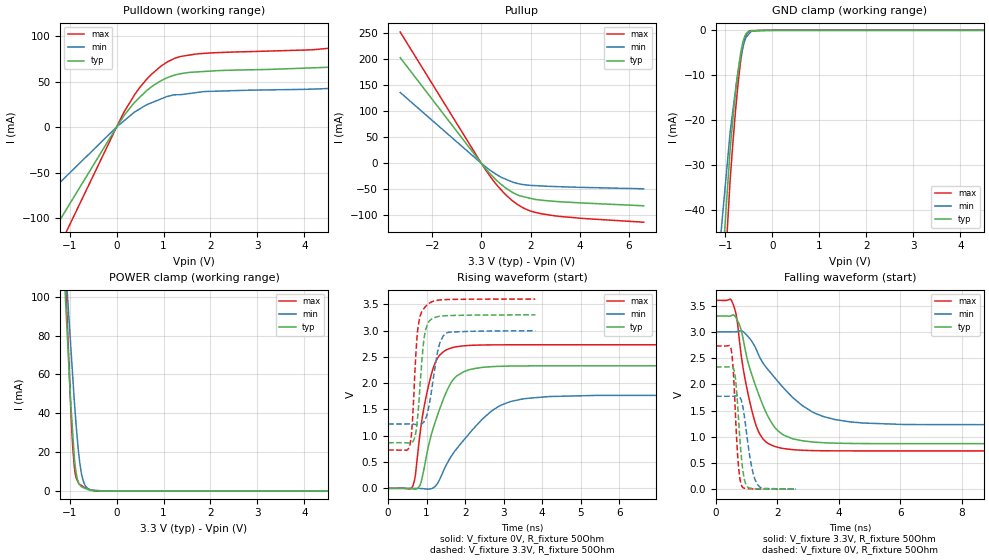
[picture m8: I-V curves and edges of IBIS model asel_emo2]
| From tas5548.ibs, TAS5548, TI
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|   asel_emo2 Model
[Model]   asel_emo2
Model_type   I/O
Polarity   Non-Inverting
Enable   Active-Low
Vinl = 0.8
Vinh = 2.0
Vmeas = 1.65
Vref = 1.65
Cref = 2pF
Rref = 50
|   typ   min   max
|   (nom PVT)   (fast PVT)   (slow PVT)
|C_comp from frequency sweep method (F=50MHz)
|Average
|C_comp   3.022e-12   2.885e-12   3.227e-12
|ON state : BUFFER OUTPUT TURNED HIGH
|C_comp   4.084e-12   3.837e-12   4.481e-12
|OFF state: BUFFER IN HIGH IMPEDANCE
|C_comp   1.959e-12   1.934e-12   1.973e-12
|C_comp from LC tank measurement(L=1nH)
|Average
|Resonant Frequency(Hz)   3.780e+09   3.820e+09   3.745e+09
C_comp   1.788e-12   1.746e-12   1.824e-12
|ON state : BUFFER OUTPUT TURNED HIGH
|Resonant Frequency(Hz)   3.590e+09   3.670e+09   3.540e+09
|C_comp   1.967e-12   1.883e-12   2.023e-12
|OFF state: BUFFER IN HIGH IMPEDANCE
|Resonant Frequency(Hz)   3.970e+09   3.970e+09   3.950e+09
|C_comp   1.609e-12   1.609e-12   1.625e-12
| Where nom  PVT is Nominal Process, 3.3V, 27C
|   Fast PVT is Strong Process,  3.6V, 0C
|   Slow PVT is Weak Process,   3V, 125C
[Voltage Range]   3.3   3   3.6
|Ambient Temperature   27   125   0
|Junction Temperature
[Temperature Range]   27   125   0
[Pullup Reference]   3.3   3   3.6
[Pulldown Reference]   0   0   0
[Power Clamp Reference]   3.3   3   3.6
[GND Clamp Reference]   0   0   0
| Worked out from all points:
|   slope of the pulldown table from 0 to 0.495 V, typ, clamps not added: 15.1 ohm
|   slope of the pullup table from 0 to 0.495 V, typ, clamps not added: 18.5 ohm
|   GND clamp passes 1 mA (typ) near -0.57 V on its own axis
|   POWER clamp passes 1 mA (typ) near -0.64 V on its own axis
|   falling waveform, V_fixture 3.3V, R_fixture 50Ohm: 20-80 % time 825ps typ, 1.52ns min, 530ps max; typ from 3.3 V to 0.868 V
|   rising waveform, V_fixture 0V, R_fixture 50Ohm: 20-80 % time 574ps typ, 1.15ns min, 377ps max; typ from 0 V to 2.33 V
|   rising waveform, V_fixture 3.3V, R_fixture 50Ohm: 20-80 % time 160ps typ, 234ps min, 137ps max; typ from 0.868 V to 3.3 V
|   falling waveform, V_fixture 0V, R_fixture 50Ohm: 20-80 % time 180ps typ, 271ps min, 146ps max; typ from 2.33 V to 0.001 V
[Pulldown]
|   Voltage   I(typ)   I(min)   I(max)
-3.3V     -279.4mA   -166.6mA   -355.3mA
-3mV      -254uA     -151.5uA   -323uA
396mV     27.87mA    16.95mA    36.54mA
633.6mV   39.82mA    24.42mA    52.19mA
939.6mV   50.83mA    30.86mA    66.82mA
1.246V    57.38mA    35.55mA    75.8mA
2.012V    61.64mA    39.34mA    81.57mA
4.496V    65.86mA    42.46mA    86.57mA
5.148V    71.83mA    45.78mA    94.35mA
5.683V    83.14mA    53.28mA    109.3mA
6.158V    100.8mA    61.11mA    132.7mA
6.6V      125.8mA    68.39mA    165.9mA
[GND Clamp]
|   Voltage   I(typ)   I(min)   I(max)
-3.3V     -1.778A    -1.524A    -1.887A
-1.541V   -126.4mA   -96.67mA   -150.3mA
-897.6mV  -26.31mA   -22.59mA   -33.19mA
-781.2mV  -13.71mA   -13.03mA   -17.57mA
-745.8mV  -10.3mA    -10.43mA   -13.65mA
-680.4mV  -5.477mA   -6.379mA   -7.311mA
-633.6mV  -2.893mA   -4.052mA   -4.02mA
-594mV    -1.494mA   -2.491mA   -2.107mA
-501.6mV  -194.8uA   -859.2uA   -291.9uA
-447mV    -173.5uA   -202.3uA   -71.12uA
-285mV    -110.1uA   -4.856uA   -22.59uA
6.6V      0A         0A         0A
[Pullup]
|   Voltage   I(typ)   I(min)   I(max)
-3.3V     202.8mA    136mA      252mA
172.8mV   -10.2mA    -6.711mA   -12.67mA
633.6mV   -33.41mA   -22.08mA   -42.05mA
939.6mV   -45.58mA   -29.5mA    -58.02mA
1.278V    -56mA      -36.2mA    -72.4mA
1.554V    -62.22mA   -39.6mA    -81.42mA
1.912V    -66.26mA   -41.93mA   -90.08mA
2.473V    -70.87mA   -43.52mA   -97.08mA
4.162V    -76.22mA   -46.24mA   -105.9mA
6.6V      -81.49mA   -48.89mA   -113mA
[POWER Clamp]
|   Voltage   I(typ)   I(min)   I(max)
-3.3V     1.395A     1.114A     1.887A
-1.102V   106.5mA    123.6mA    124.7mA
-1.066V   88.72mA    108.7mA    98.38mA
-1.062V   86.97mA    107.2mA    95.95mA
-964.8mV  41.64mA    71.01mA    37mA
-932.4mV  29.76mA    58.94mA    22.55mA
-896.4mV  16.74mA    45.55mA    11.95mA
-838.2mV  6.354mA    27.85mA    5.522mA
-753mV    2.339mA    9.743mA    2.929mA
-678mV    1.424mA    3.257mA    1.729mA
-590.7mV  510.1uA    900.1uA    866.7uA
6.6V      0A         0A         0A
[Ramp]
R_load = 50
|   typ   min   max
dV/dt_r   1.39856/5.73678e-10   1.06271/1.14379e-09   1.63831/3.76719e-10
dV/dt_f   1.45945/8.22129e-10   1.06579/1.51855e-09   1.72222/5.29784e-10
[Falling Waveform]
V_fixture = 3.3V
V_fixture_min = 3V
V_fixture_max = 3.6V
R_fixture = 50Ohm
|   Time   V(typ)   V(min)   V(max)
0s        3.3V       3V         3.6V
540ps     3.319V     2.999V     3.553V
684ps     3.232V     3.004V     3.234V
808ps     3.058V     3.02V      2.613V
1.256ns   2.027V     2.732V     1.308V
1.52ns    1.612V     2.415V     965.6mV
1.924ns   1.172V     2.118V     813mV
3.132ns   900.7mV    1.475V     736mV
4.36ns    872.3mV    1.284V     730.1mV
15ns      867.6mV    1.224V     729.6mV
[Rising Waveform]
V_fixture = 0V
V_fixture_min = 0V
V_fixture_max = 0V
R_fixture = 50Ohm
|   Time   V(typ)   V(min)   V(max)
0s        881pV      41.41nV    657.3pV
644ps     -10.36mV   976uV      47.8mV
708ps     -15.49mV   1.28mV     246.8mV
844ps     87.85mV    -2.649mV   1.12V
1.144ns   1.074V     -873.5uV   2.22V
1.344ns   1.517V     175.5mV    2.535V
1.692ns   2.068V     666.9mV    2.68V
2.692ns   2.315V     1.473V     2.728V
3.612ns   2.329V     1.711V     2.73V
15ns      2.331V     1.771V     2.731V
[Rising Waveform]
V_fixture = 3.3V
V_fixture_min = 3V
V_fixture_max = 3.6V
R_fixture = 50Ohm
|   Time   V(typ)   V(min)   V(max)
0s        867.6mV    1.224V     729.6mV
560ps     858.9mV    1.225V     803.4mV
628ps     877.9mV    1.223V     1.221V
724ps     1.074V     1.214V     2.573V
772ps     1.387V     1.209V     3.026V
904ps     2.657V     1.241V     3.394V
972ps     3V         1.322V     3.458V
1.296ns   3.267V     2.633V     3.579V
1.476ns   3.282V     2.932V     3.589V
3.824ns   3.3V       2.998V     3.6V
[Falling Waveform]
V_fixture = 0V
V_fixture_min = 0V
V_fixture_max = 0V
R_fixture = 50Ohm
|   Time   V(typ)   V(min)   V(max)
0s        2.331V     1.771V     2.731V
496ps     2.338V     1.771V     2.655V
564ps     2.31V      1.771V     2.257V
632ps     2.12V      1.777V     1.449V
736ps     1.321V     1.77V      419mV
840ps     532.5mV    1.662V     59.69mV
1.016ns   49.42mV    972.5mV    12mV
1.204ns   12.43mV    314.4mV    6.535mV
1.348ns   7.887mV    90.47mV    4.752mV
2.604ns   1.142mV    2.712mV    559.3uV
